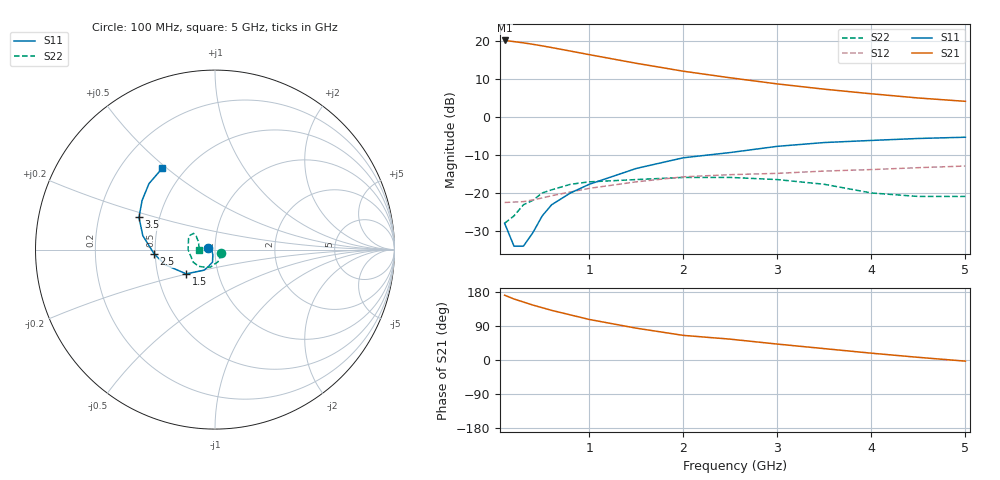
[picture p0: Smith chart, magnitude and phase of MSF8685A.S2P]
!  MSF-8685 S PARAMETERS
!  Id=16mA  LAST UPDATED 07-27-92
# ghz s ma r 50
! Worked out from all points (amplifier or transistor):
!   16 points, 100 MHz to 5 GHz, reference 50 ohm
!   highest |S21| = 20.1 dB at 100 MHz (marker M1)
!   |S21| within 3 dB of that: start of sweep to 845.2 MHz
!   unconditionally stable (mu >= 1): start of sweep to end of sweep
!   at 300 MHz: K = 1.05, MAG = 19.5 dB, |S12| = -22.3 dB
!   at 1.5 GHz: K = 1.00, MAG = 15.2 dB, |S12| = -17.1 dB
!   at 5 GHz: K = 1.13, MAG = 6.3 dB, |S12| = -12.9 dB
!   S11 on the Smith chart (normalised r, x): 100 MHz: 0.92, +0.01; 1.5 GHz: 0.70, -0.20; 2.5 GHz: 0.49, -0.03; 3.5 GHz: 0.38, +0.17; 5 GHz: 0.38, +0.48
0.1  0.04 171.0  10.09 171.0  0.075 5.0  0.04 -30.0
0.2  0.02 -180.0  9.75 161.0  0.076 10.0  0.05 -56.0
0.3  0.02 -143.0  9.38 153.0  0.077 15.0  0.07 -76.0
0.4  0.03 -113.0  8.99 145.0  0.081 17.0  0.08 -91.0
0.5  0.05 -105.0  8.57 138.0  0.086 21.0  0.1 -104.0
0.6  0.07 -101.0  8.14 131.0  0.092 25.0  0.11 -116.0
0.8  0.1 -111.0  7.32 119.0  0.103 28.0  0.13 -134.0
1  0.13 -118.0  6.57 107.0  0.115 28.0  0.14 -150.0
1.5  0.21 -140.0  5.06 84.0  0.14 28.0  0.15 180.0
2  0.29 -163.0  3.98 65.0  0.163 26.0  0.16 157.0
2.5  0.34 -176.0  3.26 55.0  0.174 28.0  0.16 150.0
3  0.41 169.0  2.71 42.0  0.181 25.0  0.15 143.0
3.5  0.46 157.0  2.31 30.0  0.194 22.0  0.13 144.0
4  0.49 146.0  2.01 18.0  0.203 20.0  0.1 156.0
4.5  0.52 135.0  1.77 7.0  0.215 17.0  0.09 173.0
5  0.54 123.0  1.6 -3.0  0.226 15.0  0.09 -178.0
